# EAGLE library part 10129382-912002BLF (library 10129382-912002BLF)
Connector Header Through Hole, Right Angle 12 position 0.100" (2.54mm) Source: Datasheet
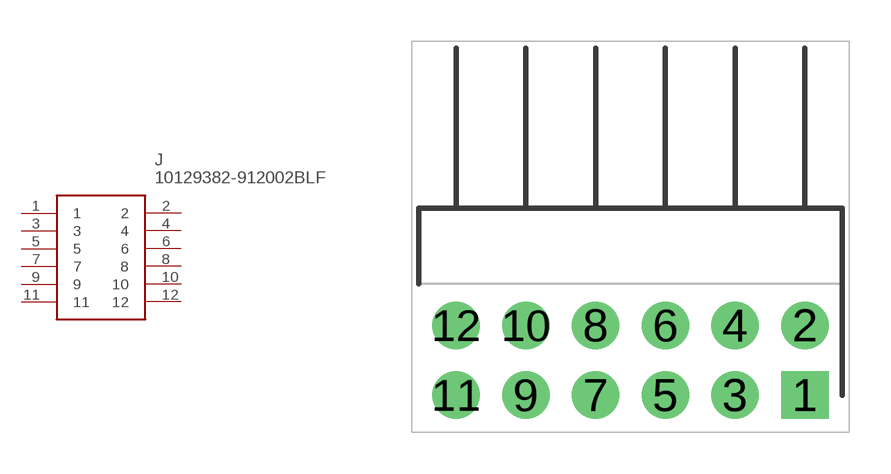
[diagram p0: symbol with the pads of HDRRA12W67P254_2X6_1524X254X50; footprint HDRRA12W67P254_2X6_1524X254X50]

Designator prefix J

## 10129382-912002BLF (Description: Connector Header Through Hole, Right Angle 12 position 0.100" (2.54mm); Height: 5.03mm; Manufacturer_Name: Amphenol; Manufacturer_Part_Number: 10129382-912002BLF)  [HDRRA12W67P254_2X6_1524X254X50]
1  1
2  2
3  3
4  4
5  5
6  6
7  7
8  8
9  9
10  10
11  11
12  12

## Footprint HDRRA12W67P254_2X6_1524X254X50 (pad centres in mm)
10129382-912002BLF
drill 1.15 pad 1.725 square: 1 0,0
drill 1.15 pad 1.725: 2 0,2.54; 3 -2.54,0; 4 -2.54,2.54; 5 -5.08,0; 6 -5.08,2.54; 7 -7.62,0; 8 -7.62,2.54; 9 -10.16,0; 10 -10.16,2.54; 11 -12.7,0; 12 -12.7,2.54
